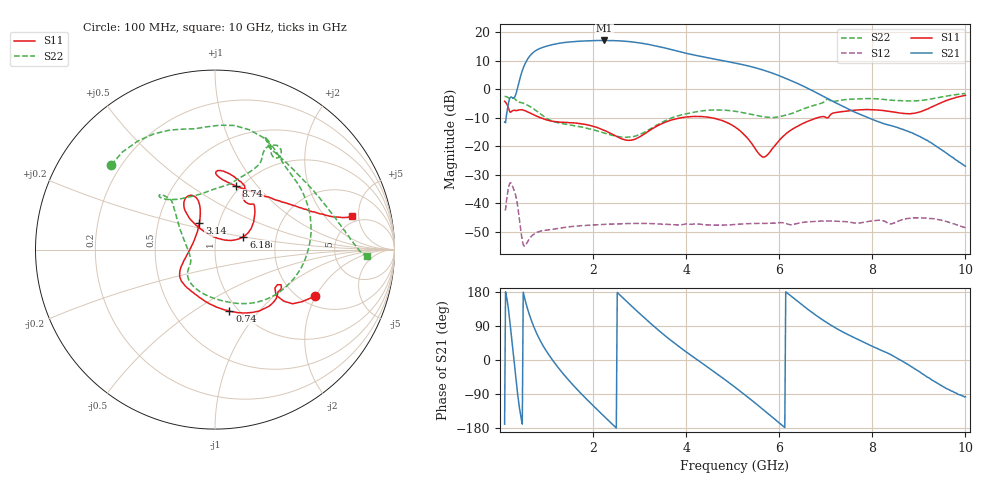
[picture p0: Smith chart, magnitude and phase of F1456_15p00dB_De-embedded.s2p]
! Integrated Device Technology
! Corporate Headquarters
! 6024 Silver Creek Valley Road
! San Jose, CA 95138  USA
! Phone:  1-408-284-8200
! Toll Free:  1-800-223-1366
! Webpage:  http://www.idt.com/
! Timing and RF Division
! 515 Groton Road, Suite 102
! Westford, MA 01886-6024
! Device:  F1456
! Description: 6-bit 0.5 dB Transmit Variable Gain Amplifier
! Frequency:  2100.0 -  2950.00 MHz
! Package:  6x6 mm Thin QFN Plastic Package: 28 pin
! State:  30
! Atten State:  15.0 dB
! Voltage:  +5.00 Volts
! Current:  217.017 mA
! Data:  The device was measured on a the F1455 evaluation board which has
!  individual transmission lines to the RF pins.  Data was collected
!  using a calibrated network analyzer.  The evaluation board was
!  de-embedded using a TRL calibration technique.
!  The reference plane is the edge of the package pin.
!  Pin  1 = CSb
!  Pin  2 = DATA
!  Pin  3 = CLK
!  Pin  4 = RSET
!  Pin  5 = GND
!  Pin  6 = RFIN  = Port 1
!  Pin  7 = GND
!  Pin  8 = NC
!  Pin  9 = NC
!  Pin 10 = NC
!  Pin 11 = NC
!  Pin 12 = NC
!  Pin 13 = NC
!  Pin 14 = /STBY
!  Pin 15 = GND
!  Pin 16 = RFOUT  = Port 2
!  Pin 17 = GND
!  Pin 18 = NC
!  Pin 19 = NC
!  Pin 20 = NC
!  Pin 21 = GND
!  Pin 22 = NC
!  Pin 23 = GND
!  Pin 24 = NC
!  Pin 25 = NC
!  Pin 26 = NC
!  Pin 27 = GND
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# GHz S dB R 50
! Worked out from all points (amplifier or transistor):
!   496 points, 100 MHz to 10 GHz, reference 50 ohm
!   highest |S21| = 17.2 dB at 2.24 GHz (marker M1)
!   |S21| within 3 dB of that: 832 MHz to 3.633 GHz (2.801 GHz wide, 125 % of centre)
!   unconditionally stable (mu >= 1): start of sweep to end of sweep
!   at 1.74 GHz: K = 15.91, MAG = 17.4 dB, |S12| = -47.9 dB
!   at 5.06 GHz: K = 32.60, MAG = 10.2 dB, |S12| = -47.5 dB
!   at 10 GHz: K = 332.92, MAG = -17.4 dB, |S12| = -48.6 dB
!   S11 on the Smith chart (normalised r, x): 100 MHz: 2.35, -1.97; 740 MHz: 0.91, -0.71; 3.14 GHz: 0.81, +0.25; 6.18 GHz: 1.36, +0.20; 8.74 GHz: 0.95, +0.78; 10 GHz: 4.22, +4.09
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0.1  -4.22 -25.1  -11.46 -169.2  -42.30 47.9  -2.55 140.8
0.32  -7.40 -32.0  -2.59 -20.4  -36.34 -146.9  -3.35 66.6
0.44  -7.17 -41.6  4.47 -142.6  -48.57 136.7  -4.59 38.2
0.58  -7.79 -59.0  10.25 140.3  -53.98 164.5  -5.46 5.7
0.74  -9.07 -76.8  13.29 83.9  -50.79 136.1  -7.03 -28.3
0.96  -10.52 -98.2  14.97 30.8  -49.58 95.1  -9.73 -66.9
1.18  -11.37 -115.3  15.90 -8.7  -49.09 69.4  -11.44 -93.6
1.48  -11.69 -131.8  16.63 -53.8  -48.35 44.3  -12.45 -119.4
1.76  -12.13 -142.6  16.96 -90.8  -47.90 25.8  -13.27 -133.9
2.24  -14.39 -158.6  17.18 -148.9  -47.49 -0.3  -15.35 -146.8
2.64  -17.54 172.5  16.97 164.1  -47.25 -20.4  -16.82 -161.0
3.14  -15.25 120.1  15.95 107.1  -47.14 -45.3  -14.74 161.8
3.4  -12.70 110.8  15.08 79.2  -47.31 -57.4  -12.34 146.1
3.74  -10.55 109.3  13.74 45.3  -47.59 -71.8  -9.75 134.6
4.08  -9.61 113.9  12.38 14.5  -47.46 -86.9  -8.35 131.9
5.06  -13.33 129.1  9.22 -72.7  -47.51 -130.2  -7.73 135.9
5.66  -23.80 73.7  6.75 -131.4  -47.11 -164.0  -9.64 118.1
6.18  -15.19 24.5  3.54 176.0  -47.36 163.3  -8.90 81.6
6.7  -10.70 40.9  -0.36 125.9  -46.50 138.0  -5.87 63.8
8.36  -7.72 88.0  -12.59 16.5  -47.22 67.0  -3.77 62.5
8.74  -8.56 71.8  -14.58 -10.1  -45.47 60.1  -4.08 49.2
10  -2.10 13.7  -27.02 -97.0  -48.64 -24.4  -1.46 -2.5
